| / 7\'7
| \ \   Xilinx Inc.
| / /
| \_\/.\   IBIS Model for Virtex-II
[IBIS ver]   2.1
[File name]   virtex2.ibs
[File Rev]   2.6
[Date]   Oct. 21, 2002
[Source]   Hspice simulations (udr4_u018_u015-33.lib)
[Notes]   Xilinx IBIS models for Virtex-II I/O's.
   COMMENTS: Models include process corners for MIN and MAX.
   See [Pin] section for details.
[Disclaimer] The data in this model is derived from SPICE simulations using
   modeling information extracted from the target process. While
   a great deal of care has been taken to provide information
   that is accurate, this model is considered preliminary as it
   has not been verified by actual silicon measurement. Treat the
   data in this model as preliminary until actual silicon
   verification is performed.
[Copyright]   Copyright 2002, Xilinx Inc., All rights reserved
|   Component Virtex-II
[Component]   VIRTEX-II
[Manufacturer]   Xilinx Inc.
[Package]
| Package Parasitics
| variable   typ   min   max
R_pkg   0.1   NA   NA
L_pkg   0.8nH   NA   NA
C_pkg   0.5pF   NA   NA
| Note: The following pin list is an EXAMPLE only.
|   The model_name is obvious and self-explanatory.
|   Please select the models accordingly.
|   The pin name is arbitrarily numbered and does not corresponds
|   to the pinout in the product package. Add the device pinout to
|   match the package type and the pinout for the particular design.
|   Please note that the DCI LVCMOS15 through LVCMOS33 models have
|   been generated for a 50 Ohms impedance.For other impedance values
|   ie 25,40,65,75 models are available. Please contact the Xilinx
|   Hotline for these models.
|   All the DCI Ibis models (TYP/MIN/MAX) have been generated for
|   specific PVT conditions. These models are good only for these
|   conditions. For details contact the Hotline.
[Pin]  signal_name   model_name   R_pin   L_pin   C_pin
|   LVTTL FAST SLEW RATE
1   LVTTL2F   LVTTL2F
2   LVTTL4F   LVTTL4F
3   LVTTL6F   LVTTL6F
4   LVTTL8F   LVTTL8F
5   LVTTL12F   LVTTL12F
6   LVTTL16F   LVTTL16F
7   LVTTL24F   LVTTL24F
|   LVTTL SLOW SLEW RATE
8   LVTTL2S   LVTTL2S
9   LVTTL4S   LVTTL4S
10   LVTTL6S   LVTTL6S
11   LVTTL8S   LVTTL8S
12   LVTTL12S   LVTTL12S
13   LVTTL16S   LVTTL16S
14   LVTTL24S   LVTTL24S
|   LVCMOS33 FAST SLEW RATE
15   LVCM32F   LVCM32F
16   LVCM34F   LVCM34F
17   LVCM36F   LVCM36F
18   LVCM38F   LVCM38F
19   LVCM312F   LVCM312F
20   LVCM316F   LVCM316F
21   LVCM324F   LVCM324F
|   LVCMOS33 SLOW SLEW RATE
22   LVCM32S   LVCM32S
23   LVCM34S   LVCM34S
24   LVCM36S   LVCM36S
25   LVCM38S   LVCM38S
26   LVCM312S   LVCM312S
27   LVCM316S   LVCM316S
28   LVCM324S   LVCM324S
|   LVCMOS25 FAST SLEW RATE
29   LVCM22F   LVCM22F
30   LVCM24F   LVCM24F
31   LVCM26F   LVCM26F
32   LVCM28F   LVCM28F
33   LVCM212F   LVCM212F
34   LVCM216F   LVCM216F
35   LVCM224F   LVCM224F
|   LVCMOS25 SLOW SLEW RATE
36   LVCM22S   LVCM22S
37   LVCM24S   LVCM24S
38   LVCM26S   LVCM26S
39   LVCM28S   LVCM28S
40   LVCM212S   LVCM212S
41   LVCM216S   LVCM216S
42   LVCM224S   LVCM224S
|   LVCMOS18 FAST SLEW RATE
43   LVCM82F   LVCM82F
44   LVCM84F   LVCM84F
45   LVCM86F   LVCM86F
46   LVCM88F   LVCM88F
47   LVCM812F   LVCM812F
48   LVCM816F   LVCM816F
|   LVCMOS18 SLOW SLEW RATE
49   LVCM82S   LVCM82S
50   LVCM84S   LVCM84S
51   LVCM86S   LVCM86S
52   LVCM88S   LVCM88S
53   LVCM812S   LVCM812S
54   LVCM816S   LVCM816S
|   LVCMOS15 FAST SLEW RATE
55   LVCM52F   LVCM52F
56   LVCM54F   LVCM54F
57   LVCM56F   LVCM56F
58   LVCM58F   LVCM58F
59   LVCM512F   LVCM512F
60   LVCM516F   LVCM516F
|   LVCMOS15 SLOW SLEW RATE
61   LVCM52S   LVCM52S
62   LVCM54S   LVCM54S
63   LVCM56S   LVCM56S
64   LVCM58S   LVCM58S
65   LVCM512S   LVCM512S
66   LVCM516S   LVCM516S
|   HSTL I-IV 1.5V
67   HSTL1_15   HSTL1_15
68   HSTL2_15   HSTL2_15
69   HSTL3_15   HSTL3_15
70   HSTL4_15   HSTL4_15
|   GTL AND GTPPLUS
71   GTL   GTL
72   GTLP   GTLP
|   SSTL18, SSTL2 AND SSTL3
73   SSTL18C1   SSTL18C1
74   SSTL18C2   SSTL18C2
75   SSTL2C1   SSTL2C1
76   SSTL2C2   SSTL2C2
77   SSTL3C1   SSTL3C1
78   SSTL3C2   SSTL3C2
|   PCI
79   PCI33   PCI33
80   PCI66   PCI66
81   PCIX   PCIX
|   AGP
82   AGP2X   AGP2X
|   LVPECL
83P   LVPECLP   LVPECL
83N   LVPECLN   LVPECL
|   LVDS25 GENERAL AND EXTENDED
84P   LVDS25P   LVDS25
84N   LVDS25N   LVDS25
85P   LVDS25EP   LVDS25E
85N   LVDS25EN   LVDS25E
|   LVDS33 GENERAL AND EXTENDED
86P   LVDS33P   LVDS33
86N   LVDS33N   LVDS33
87P   LVDS33EP   LVDS33E
87N   LVDS33EN   LVDS33E
|   LDT
88P   LDT25P   LDT25
88N   LDT25N   LDT25
|   BUSSLVDS
89P   BUSSLVDSP   BUSSLVDS
89N   BUSSLVDSN   BUSSLVDS
|   DCI HSTL I-IV 1.5V
|   INPUT MODELS
90   DCIHSTL15_I   DCIHSTL15_I
91   DCIHSTL25_I   DCIHSTL25_I
92   DCIHSTL35_I   DCIHSTL35_I
93   DCIHSTL45_I   DCIHSTL45_I
|   OUTPUT MODELS
94   DCIHSTL15_O   DCIHSTL15_O
95   DCIHSTL25_O   DCIHSTL25_O
96   DCIHSTL35_O   DCIHSTL35_O
97   DCIHSTL45_O   DCIHSTL45_O
|   DCI GTL AND GTLPLUS
|   INPUT MODELS
98   DCIGTL_I   DCIGTL_I
99   DCIGTLP_I   DCIGTLP_I
|   OUTPUT MODELS
100   DCIGTL_O   DCIGTL_O
101   DCIGTLP_O   DCIGTLP_O
|   DCI SSTL18, SSTL2 AND SSTL3
|   INPUT MODELS
102   DCISSTL18C1_I   DCISSTL18C1_I
103   DCISSTL18C2_I   DCISSTL18C2_I
104   DCISSTL2C1_I   DCISSTL2C1_I
105   DCISSTL2C2_I   DCISSTL2C2_I
106   DCISSTL3C1_I   DCISSTL3C1_I
107   DCISSTL3C2_I   DCISSTL3C2_I
|   OUTPUT MODELS
108   DCISSTL18C1_O   DCISSTL18C1_O
109   DCISSTL18C2_O   DCISSTL18C2_O
110   DCISSTL2C1_O   DCISSTL2C1_O
111   DCISSTL2C2_O   DCISSTL2C2_O
112   DCISSTL3C1_O   DCISSTL3C1_O
113   DCISSTL3C2_O   DCISSTL3C2_O
|   DCI LVCMOS15 THRU LVCMOS33 50 Ohms impedance
114   DCILVCMOS15_50   DCILVCMOS15_50
115   DCILVCMOS18_50   DCILVCMOS18_50
116   DCILVCMOS25_50   DCILVCMOS25_50
117   DCILVCMOS33_50   DCILVCMOS33_50
|   DCI LVCMOS15 THRU LVCMOS33 DRIVER/2 25 Ohms impedance
118   DCILVCMOS15DV2_50   DCILVCMOS15DV2_50
119   DCILVCMOS18DV2_50   DCILVCMOS18DV2_50
120   DCILVCMOS25DV2_50   DCILVCMOS25DV2_50
121   DCILVCMOS33DV2_50   DCILVCMOS33DV2_50
|   HSTL CLASSI-IV 1.8V
122   HSTL1_18   HSTL1_18
123   HSTL2_18   HSTL2_18
124   HSTL3_18   HSTL3_18
125   HSTL4_18   HSTL4_18
|   DCI HSTL I-IV 1.8V
|   INPUT MODELS
126   DCIHSTL18_I   DCIHSTL18_I
127   DCIHSTL28_I   DCIHSTL28_I
128   DCIHSTL38_I   DCIHSTL38_I
129   DCIHSTL48_I   DCIHSTL48_I
|   OUTPUT MODELS
130   DCIHSTL18_O   DCIHSTL18_O
131   DCIHSTL28_O   DCIHSTL28_O
132   DCIHSTL38_O   DCIHSTL38_O
133   DCIHSTL48_O   DCIHSTL48_O
|   LVDS receiver models with internal termination.
134   DCILVDS25   DCILVDS25
135   DCILVDS25E   DCILVDS25E
PGND   GND   GND
VCCO   VCCO   POWER
[Diff Pin]   inv_pin   vdiff   tdelay_typ   tdelay_min   tdelay_max
| Here is just a sample format for differential pin pairs.
| Edit the list based on your applications.
83P   83N   850mV   0   0   0
84P   84N   350mV   0   0   0
85P   85N   630mV   0   0   0
86P   86N   350mV   0   0   0
87P   87N   630mV   0   0   0
88P   88N   600mV   0   0   0
89P   89N   350mV   0   0   0
| Models and submodels in the file (135): LVTTL2F (I/O), LVTTL4F (I/O), LVTTL6F (I/O), LVTTL8F (I/O), LVTTL12F (I/O), LVTTL16F (I/O), LVTTL24F (I/O), LVTTL2S (I/O), LVTTL4S (I/O), LVTTL6S (I/O), LVTTL8S (I/O), LVTTL12S (I/O), LVTTL16S (I/O), LVTTL24S (I/O), LVCM32F (I/O), LVCM34F (I/O), LVCM36F (I/O), LVCM38F (I/O), LVCM312F (I/O), LVCM316F (I/O), LVCM324F (I/O), LVCM32S (I/O), LVCM34S (I/O), LVCM36S (I/O), LVCM38S (I/O), LVCM312S (I/O), LVCM316S (I/O), LVCM324S (I/O), LVCM22F (I/O), LVCM24F (I/O), LVCM26F (I/O), LVCM28F (I/O), LVCM212F (I/O), LVCM216F (I/O), LVCM224F (I/O), LVCM22S (I/O), LVCM24S (I/O), LVCM26S (I/O), LVCM28S (I/O), LVCM212S (I/O), LVCM216S (I/O), LVCM224S (I/O), LVCM82F (I/O), LVCM84F (I/O), LVCM86F (I/O), LVCM88F (I/O), LVCM812F (I/O), LVCM816F (I/O), LVCM82S (I/O), LVCM84S (I/O), LVCM86S (I/O), LVCM88S (I/O), LVCM812S (I/O), LVCM816S (I/O), LVCM52F (I/O), LVCM54F (I/O), LVCM56F (I/O), LVCM58F (I/O), LVCM512F (I/O), LVCM516F (I/O), LVCM52S (I/O), LVCM54S (I/O), LVCM56S (I/O), LVCM58S (I/O), LVCM512S (I/O), LVCM516S (I/O), HSTL1_15 (I/O), HSTL2_15 (I/O), HSTL3_15 (I/O), HSTL4_15 (I/O), GTL (I/O_open_drain), GTLP (I/O_open_drain), SSTL18C1 (I/O), SSTL18C2 (I/O), SSTL2C1 (I/O), SSTL2C2 (I/O), SSTL3C1 (I/O), SSTL3C2 (I/O), PCI33 (I/O), PCI66 (I/O)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
